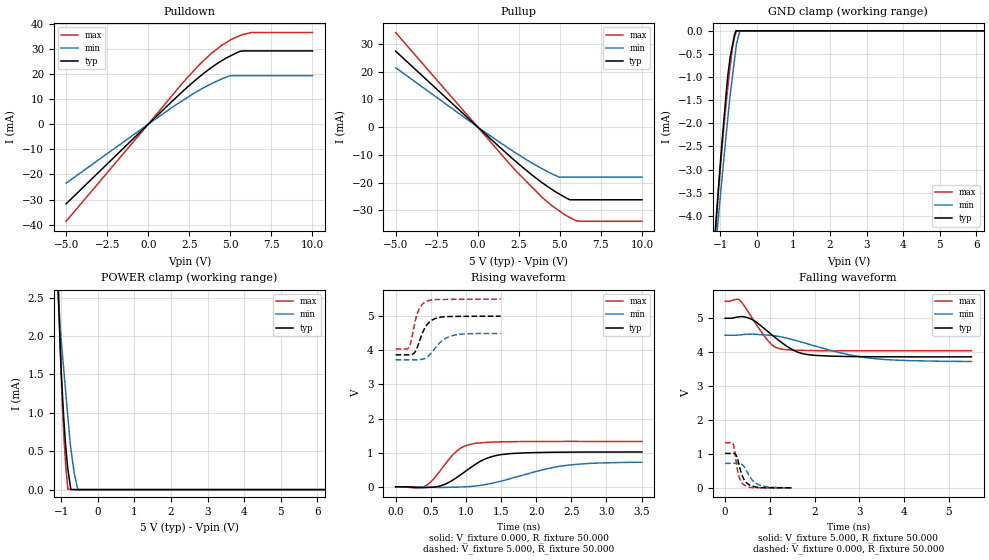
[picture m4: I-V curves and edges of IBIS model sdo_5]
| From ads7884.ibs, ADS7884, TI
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|   sdo_5 Model
[Model]   sdo_5
Model_type   3-state
Polarity   Non-Inverting
Vmeas = 2.5
Vref = 2.5
Cref = 10pF
Rref = 50
|   typ   min   max
|   (nom PVT)   (Fast PVT)   (slow PVT)
|C_comp from frequency sweep method(F=48MHz)
|C_comp   8.529e-13   8.262e-13   9.423e-13
|ON state : BUFFER OUTPUT TURNED HIGH
|C_comp   8.529e-13   8.262e-13   9.423e-13
|OFF state: BUFFER IN HIGH IMPEDANCE
|C_comp   1.112e-12   9.514e-13   1.282e-12
|C_comp from LC tank measurement(L=1nH)
|Resonant Frequency(Hz)   6.550e+09   6.740e+09   6.440e+09
C_comp   5.910e-13   5.582e-13   6.114e-13
|ON state : BUFFER OUTPUT TURNED HIGH
|Resonant Frequency(Hz)   6.550e+09   6.740e+09   6.440e+09
|C_comp   5.910e-13   5.582e-13   6.114e-13
|OFF state: BUFFER IN HIGH IMPEDANCE
|Resonant Frequency   6.100e+09   5.860e+09   6.560e+09
|C_comp   6.814e-13   5.892e-13   7.384e-13
| Where nom  PVT is Nominal Process,  5V,  30C
|   Fast PVT is Strong Process,   5.5V,  -40C
|   Slow PVT is Weak Process,   4.5V,  130C
[Voltage Range]   5   4.5   5.5
|Ambient Temperature   25   125   -40
|Junction Temperature
[Temperature Range]   30   130   -40
[Pullup Reference]   5   4.5   5.5
[Pulldown Reference]   0   0   0
[Power Clamp Reference]   5   4.5   5.5
[GND Clamp Reference]   0   0   0
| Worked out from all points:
|   slope of the pulldown table from 0 to 0.75 V, typ, clamps not added: 159 ohm
|   slope of the pullup table from 0 to 0.75 V, typ, clamps not added: 184 ohm
|   GND clamp passes 1 mA (typ) near -0.79 V on its own axis
|   POWER clamp passes 1 mA (typ) near -0.94 V on its own axis
|   falling waveform, V_fixture 5.000, R_fixture 50.000: 20-80 % time 677ps typ, 1.37ns min, 456ps max; typ from 5 V to 3.86 V
|   rising waveform, V_fixture 0.000, R_fixture 50.000: 20-80 % time 457ps typ, 810ps min, 324ps max; typ from 0 V to 1.02 V
|   rising waveform, V_fixture 5.000, R_fixture 50.000: 20-80 % time 146ps typ, 216ps min, 108ps max; typ from 3.87 V to 5 V
|   falling waveform, V_fixture 0.000, R_fixture 50.000: 20-80 % time 158ps typ, 231ps min, 114ps max; typ from 1.02 V to 0 V
[Pulldown]
|   Voltage   I(typ)   I(min)   I(max)
-5V       -31.67mA   -23.44mA   -38.63mA
0V        0A         0A         0A
2.365V    14.63mA    10.56mA    18.41mA
3.146V    19.01mA    13.67mA    23.89mA
3.844V    22.53mA    16.1mA     28.17mA
4.476V    25.28mA    18mA       31.39mA
4.968V    27.05mA    19.23mA    33.37mA
5.61V     29.05mA    19.33mA    35.32mA
6.253V    29.16mA    19.33mA    36.46mA
10V       29.16mA    19.33mA    36.46mA
[GND Clamp]
|   Voltage   I(typ)   I(min)   I(max)
-5V       -53.57mA   -43.19mA   -66.66mA
-1.15V    -4.501mA   -4.926mA   -4.646mA
-1.036V   -3.282mA   -3.931mA   -3.369mA
-891.5mV  -1.873mA   -2.71mA    -2.019mA
-785mV    -934.7uA   -1.843mA   -1.185mA
-725mV    -567.7uA   -1.38mA    -769.3uA
-660.5mV  -300.2uA   -966.2uA   -355.8uA
-610mV    -90.75uA   -642uA     -151.9uA
-570mV    0A         -385.1uA   -42.82uA
-554mV    0A         -282.4uA   -4.619uA
-459.5mV  0A         0A         -3.83uA
10V       0A         0A         0A
[Pullup]
|   Voltage   I(typ)   I(min)   I(max)
-5V       27.37mA    21.4mA     34.07mA
0V        0A         0A         0A
2.315V    -12.39mA   -9.318mA   -15.74mA
3.965V    -20.24mA   -15.17mA   -25.59mA
4.537V    -22.58mA   -16.92mA   -28.44mA
4.941V    -24.04mA   -18.02mA   -30.12mA
5.61V     -26.22mA   -18.04mA   -32.61mA
5.995V    -26.22mA   -18.04mA   -33.82mA
10V       -26.22mA   -18.04mA   -33.98mA
[POWER Clamp]
|   Voltage   I(typ)   I(min)   I(max)
-5V       75.39mA    59.43mA    93.42mA
-1.13V    3.198mA    2.894mA    3.781mA
-1.036V   1.987mA    2.179mA    2.042mA
-1.024V   1.844mA    2.104mA    1.821mA
-990.5mV  1.474mA    1.899mA    1.387mA
-930mV    940.5uA    1.568mA    737.4uA
-869.5mV  536uA      1.238mA    275.8uA
-814.5mV  260.2uA    938.7uA    4.487uA
-735mV    510.5nA    535.5uA    2.395uA
-644mV    138.9nA    215.4uA    0A
-545mV    0A         0A         0A
10V       0A         0A         0A
[Ramp]
R_load = 50
|   typ   min   max
dV/dt_r   0.60942/4.54178e-10   0.439094/8.28206e-10   0.793079/3.2211e-10
dV/dt_f   0.679926/6.73287e-10   0.475369/1.39155e-09   0.86899/4.52328e-10
[Falling Waveform]
V_fixture = 5.000
V_fixture_min = 4.500
V_fixture_max = 5.500
R_fixture = 50.000
|  time   V(typ)   V(min)   V(max)
0s        5V         4.5V       5.5V
330ps     5.045V     4.509V     5.527V
605ps     4.961V     4.534V     5.003V
930ps     4.637V     4.505V     4.384V
1.08ns    4.474V     4.487V     4.184V
1.255ns   4.293V     4.449V     4.091V
1.605ns   4.01V      4.336V     4.058V
1.98ns    3.909V     4.193V     4.047V
3.405ns   3.865V     3.801V     4.041V
5.505ns   3.863V     3.724V     4.045V
[Rising Waveform]
V_fixture = 0.000
V_fixture_min = 0.000
V_fixture_max = 0.000
R_fixture = 50.000
|  time   V(typ)   V(min)   V(max)
0s        34.24uV    13.05uV    66.83uV
280ps     -17.12mV   -675.1uV   -31.84mV
430ps     -23.34mV   -9.922mV   32.05mV
655ps     38.45mV    -20.99mV   526.1mV
880ps     287mV      -9.279mV   1.063V
1.105ns   615mV      16.04mV    1.264V
1.33ns    858.1mV    85.33mV    1.305V
1.63ns    970.8mV    236.9mV    1.321V
2.405ns   1.014V     621.5mV    1.33V
3.505ns   1.02V      720.2mV    1.328V
[Rising Waveform]
V_fixture = 5.000
V_fixture_min = 4.500
V_fixture_max = 5.500
R_fixture = 50.000
|  time   V(typ)   V(min)   V(max)
0s        3.868V     3.72V      4.041V
190ps     3.868V     3.72V      4.085V
220ps     3.874V     3.72V      4.266V
265ps     3.922V     3.72V      4.728V
315ps     4.126V     3.723V     5.114V
365ps     4.42V      3.733V     5.311V
440ps     4.734V     3.792V     5.436V
570ps     4.936V     4.084V     5.486V
780ps     4.991V     4.413V     5.493V
1.495ns   5V         4.493V     5.5V
[Falling Waveform]
V_fixture = 0.000
V_fixture_min = 0.000
V_fixture_max = 0.000
R_fixture = 50.000
|  time   V(typ)   V(min)   V(max)
0s        1.016V     722.6mV    1.331V
175ps     1.019V     722.5mV    1.304V
200ps     1.016V     722.6mV    1.186V
240ps     976.9mV    723.1mV    830.6mV
305ps     713.8mV    720.1mV    360.5mV
370ps     402.9mV    694.1mV    162.1mV
435ps     219.5mV    603.6mV    76.39mV
610ps     50.69mV    227.2mV    6.891mV
775ps     10.97mV    79.6mV     1.923mV
1.495ns   0V         3.847mV    0V
